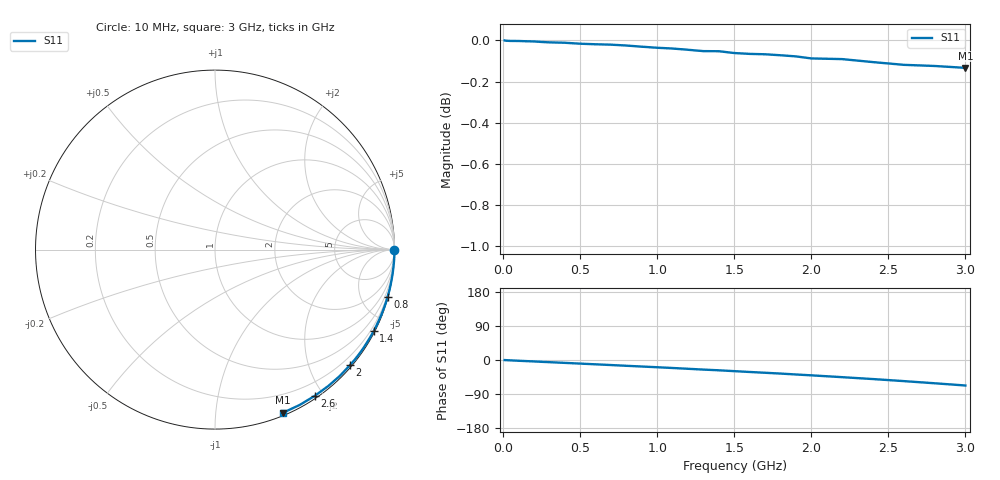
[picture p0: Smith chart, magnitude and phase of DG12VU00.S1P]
! SIEMENS Small Signal Semiconductors
! BAV70
! Silicon Switching Diode in SOT23
! VR = 12 V
! S-Parameters:  May  1995
# GHz  S  MA  R  50
!  f  S11
! GHz  MAG  ANG
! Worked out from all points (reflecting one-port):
!   30 points, 10 MHz to 3 GHz, reference 50 ohm
!   lowest |S11| = -0.1 dB at 3 GHz (marker M1), VSWR 130.32, Z = 1.25 - j75.1 ohm
!   phase of S11 starts at -0 deg and turns -67 deg over the sweep
!   S11 on the Smith chart (normalised r, x): 10 MHz: open; 800 MHz: 0.08, -7.44; 1.4 GHz: 0.05, -4.13; 2 GHz: 0.04, -2.71; 2.6 GHz: 0.03, -1.89; 3 GHz: 0.02, -1.50
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0.01  1 -0.2
0.1  0.9997 -2.0
0.15  0.9995 -2.9
0.2  0.9994 -3.8
0.25  0.9991 -4.8
0.3  0.9989 -5.7
0.4  0.9987 -7.6
0.5  0.9982 -9.5
0.6  0.9979 -11.4
0.7  0.9976 -13.3
0.8  0.9972 -15.3
0.9  0.9965 -17.2
1  0.9959 -19.1
1.1  0.9955 -21.1
1.2  0.9948 -23.2
1.3  0.994 -25.3
1.4  0.994 -27.2
1.5  0.993 -29.4
1.6  0.9925 -31.6
1.7  0.9923 -33.7
1.8  0.9917 -35.8
1.9  0.9911 -38.2
2  0.99 -40.5
2.2  0.9896 -45.3
2.4  0.9879 -50.3
2.6  0.9864 -55.7
2.8  0.9858 -61.4
3  0.9848 -67.3
